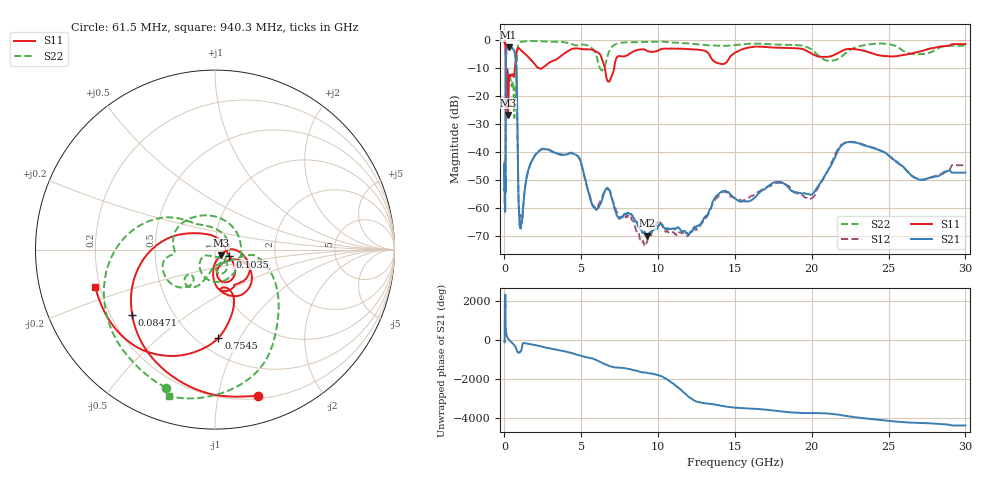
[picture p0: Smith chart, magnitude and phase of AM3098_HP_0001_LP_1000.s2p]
! Date/Time: Thu, Feb 28, 2019 8:32 AM
! Network Analyzer: Agilent Technologies E8364B Rev: A.07.50.67
! Sweep from 0.010 to 30.000 GHz, 1601 Points, Sweep Type: LOG
! Power Supply: 5.022 V, 0.002 A
# Hz S DB R 50
!freq MagS11 AngS11 MagS21 AngS21 MagS12 AngS12 MagS22 AngS22
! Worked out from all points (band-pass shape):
!   1601 points, 10 MHz to 30 GHz, reference 50 ohm
!   highest |S21| = -2.73 dB at 266.5 MHz (marker M1); lowest = -69.9 dB at 9.302 GHz (marker M2)
!   |S21| within 3 dB of the highest: 105.6 MHz to 705.9 MHz (600.3 MHz wide, 148 % of centre)
!   lowest |S11| = -26.9 dB at 233.9 MHz (marker M3), VSWR 1.10, Z = 53.2 - j3.4 ohm
!   |S11| at or under -10 dB: 91.05 MHz to 682.5 MHz (591.4 MHz wide, 153 % of centre); 2.158 GHz to 2.516 GHz (358.2 MHz wide, 15.3 % of centre); 6.528 GHz to 7.149 GHz (621.5 MHz wide, 9.09 % of centre)
!   |S22| runs from -28.0 to -0.5 dB; largest |S21 - S12| = 0.012
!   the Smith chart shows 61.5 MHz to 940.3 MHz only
!   S11 on the Smith chart (normalised r, x): 61.5 MHz: 0.23, -1.32; 84.71 MHz: 0.29, -0.32; 103.5 MHz: 1.17, -0.09; 754.5 MHz: 0.63, -0.82; 940.3 MHz: 0.18, -0.15
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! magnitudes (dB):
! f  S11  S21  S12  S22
! 10 MHz  -0.3  -44.9  -43.2  -0.6
! 38.04 MHz  -0.5  -61.1  -60.0  -0.9
! 61.5 MHz  -1.4  -53.2  -51.8  -1.8
! 73.27 MHz  -2.2  -51.3  -50.2  -2.6
! 84.71 MHz  -4.6  -28.5  -28.6  -5.2
! 103.5 MHz  -21.0  -6.1  -6.1  -15.1
! 144.7 MHz  -14.9  -3.4  -3.3  -12.8
! 233.9 MHz  -26.9  -2.8  -2.8  -12.7
! 266.5 MHz  -17.7  -2.7  -2.7  -13.0
! 550.5 MHz  -12.7  -3.4  -3.4  -14.9
! 639.6 MHz  -12.7  -4.1  -4.0  -28.0
! 754.5 MHz  -6.2  -8.7  -8.7  -19.4
! 940.3 MHz  -3.1  -60.7  -60.2  -1.3
! 1.115 GHz  -4.0  -64.7  -65.4  -0.8
! 2.084 GHz  -9.6  -40.7  -40.6  -0.6
! 4.64 GHz  -3.2  -41.1  -41.1  -2.1
! 5.812 GHz  -3.9  -59.7  -59.5  -3.8
! 7.926 GHz  -5.8  -62.3  -62.8  -1.0
! 9.302 GHz  -4.1  -69.9  -71.8  -0.9
! 19.7 GHz  -4.1  -55.0  -56.6  -2.7
! 22.67 GHz  -3.4  -36.7  -36.5  -3.2
! 30 GHz  -1.6  -47.5  -44.8  -2.2
